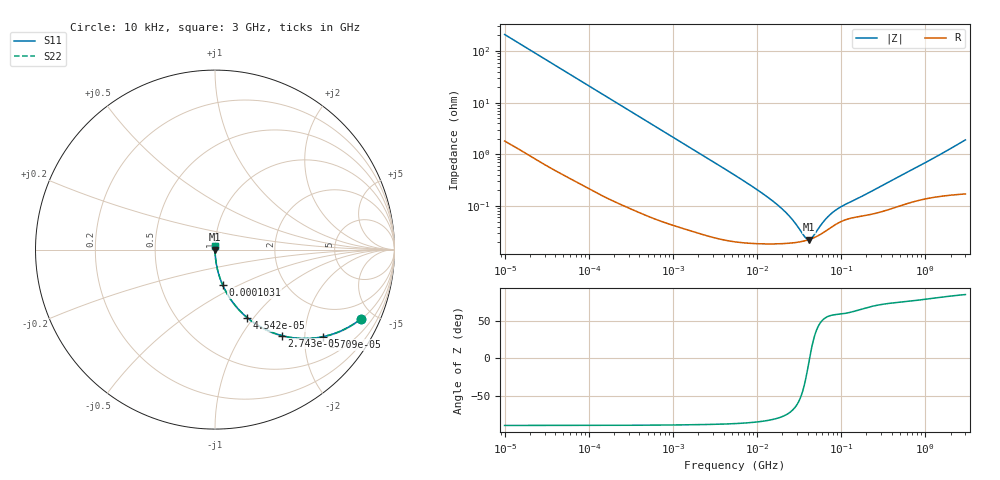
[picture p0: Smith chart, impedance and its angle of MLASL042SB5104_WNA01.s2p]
! MLASL042SB5104_WNA01  S-PARAMETER MODEL  ( Standard Model )
! Model Generated by TAIYO YUDEN Corporation (http://www.ty-top.com)
! Version 1.0
! TAIYO YUDEN Control No. 220901
! Copyright(c) 2022 TAIYO YUDEN CO.,LTD. All Rights Reserved.
! Product Description (link to TY-COMPAS)
! https://ds.yuden.co.jp/TYCOMPAS/or/detail?pn=MLASL042SB5104MWNA01&u=M
! Products Name : Multilayer Ceramic Capacitors
! Characteristics :
!  Capacitance : 0.1 [uF] , Rated Voltage : 10 [V] , TCC : X5R
!  Case Size : 0.4 x 0.2 / 0.016 x 0.008 [mm/inch] , Thickness : 0.2 / 0.008 [mm/inch]
!  (Conditions: Temperature = 25 [degC] , DC Bias Voltage = 0 [V])
! External Node Assignments :
!  1  o---| |---o  2
! GND o---------o GND
! Frequency Range : 10kHz  -  3GHz  [ 401 STEP ]
# MHZ S RI R 50
! Freq[MHz].  S11 Real  S11 Imag  S21 Real  S21 Imag  S12 Real  S12 Imag  S22 Real  S22 Imag
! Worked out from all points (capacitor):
!   401 points, 10 kHz to 3 GHz, reference 50 ohm
!   read as one part in series: C = 75.9 nF near 10.65 kHz
!   lowest |Z| = 22.4 mohm at 41.2 MHz (marker M1)
!   series resonance near 42.22 MHz, so ESL is about 190 pH
!   S11 on the Smith chart (normalised r, x): 10 kHz: 1.04, -4.19; 17.09 kHz: 1.02, -2.46; 27.43 kHz: 1.01, -1.54; 45.42 kHz: 1.01, -0.93; 103.1 kHz: 1.00, -0.41; 3 GHz: 1.00, +0.04
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0.01  0.8121 -0.3863  0.1879 0.3863  0.1879 0.3863  0.8121 -0.3863
0.01247  0.7368 -0.436  0.2632 0.436  0.2632 0.436  0.7368 -0.436
0.017091  0.6007 -0.4853  0.3993 0.4853  0.3993 0.4853  0.6007 -0.4853
0.021312  0.4933 -0.4955  0.5067 0.4955  0.5067 0.4955  0.4933 -0.4955
0.027426  0.3719 -0.4789  0.6281 0.4789  0.6281 0.4789  0.3719 -0.4789
0.045421  0.1799 -0.3795  0.8201 0.3795  0.8201 0.3795  0.1799 -0.3795
0.082683  0.0637 -0.2393  0.9363 0.2393  0.9363 0.2393  0.0637 -0.2393
0.103102  0.0425 -0.1966  0.9575 0.1966  0.9575 0.1966  0.0425 -0.1966
0.234035  0.00928 -0.0901  0.9907 0.0901  0.9907 0.0901  0.00928 -0.0901
0.683653  0.00151 -0.0313  0.9985 0.0313  0.9985 0.0313  0.00151 -0.0313
5.477226  0.000217 -0.00392  0.9998 0.00392  0.9998 0.00392  0.000217 -0.00392
11.31085  0.000188 -0.0018  0.9998 0.0018  0.9998 0.0018  0.000188 -0.0018
18.15044  0.000186 -0.000985  0.9998 0.000985  0.9998 0.000985  0.000186 -0.000985
25.67485  0.000192 -0.000539  0.9998 0.000539  0.9998 0.000539  0.000192 -0.000539
37.4819  0.000213 -0.000124  0.9998 0.000124  0.9998 0.000124  0.000213 -0.000124
41.20027  0.000222 -2.54e-05  0.9998 2.54e-05  0.9998 2.54e-05  0.000222 -2.54e-05
45.28751  0.000235 7.29e-05  0.9998 -7.29e-05  0.9998 -7.29e-05  0.000235 7.29e-05
64.06182  0.000319 0.000429  0.9997 -0.000429  0.9997 -0.000429  0.000319 0.000429
85.08137  0.000433 0.000695  0.9996 -0.000695  0.9996 -0.000695  0.000433 0.000695
106.0924  0.000521 0.000879  0.9995 -0.000879  0.9995 -0.000879  0.000521 0.000879
374.4521  0.000866 0.00283  0.9991 -0.00283  0.9991 -0.00283  0.000866 0.00283
3000  0.00206 0.0189  0.9979 -0.0189  0.9979 -0.0189  0.00206 0.0189
